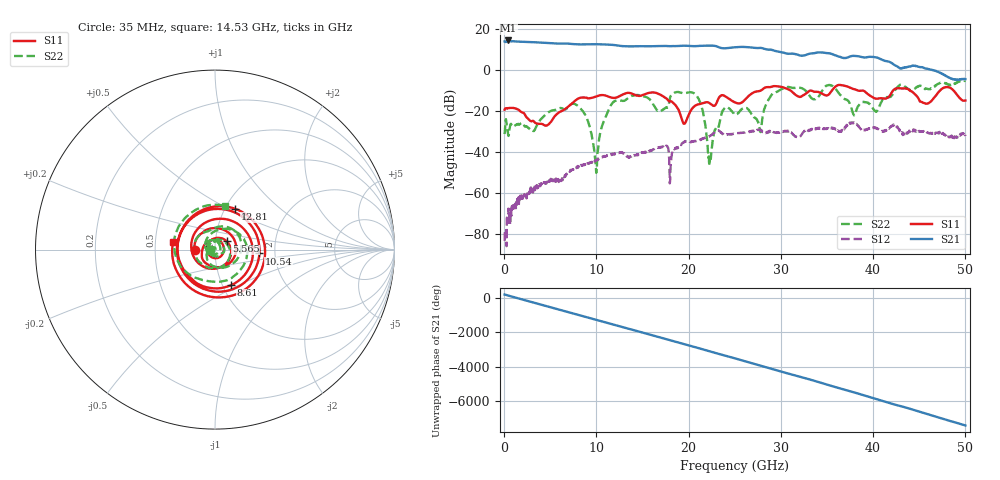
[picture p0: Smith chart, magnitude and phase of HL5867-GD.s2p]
! 4/14/2021 8:59:28 AM
! H:\PRODUCTION_DATA\TEMP_S2P.S2P
! CHANNEL.1
! TR.MEASUREMENT
! CORRECTED.DATA
# GHZ S RI R 50.0
! FREQ.GHZ  S11RE  S11IM  S21RE  S21IM  S12RE  S12IM  S22RE  S22IM
!; PortSelection: Port_12
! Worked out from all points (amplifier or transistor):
!   1429 points, 35 MHz to 50.02 GHz, reference 50 ohm
!   highest |S21| = 14.6 dB at 420 MHz (marker M1)
!   |S21| within 3 dB of that: start of sweep to 23.12 GHz
!   unconditionally stable (mu >= 1): start of sweep to end of sweep
!   at 8.365 GHz: K = 22.97, MAG = 12.9 dB, |S12| = -46.4 dB
!   at 25.02 GHz: K = 4.65, MAG = 11.4 dB, |S12| = -30.8 dB
!   at 50.02 GHz: K = 21.93, MAG = -2.5 dB, |S12| = -32.1 dB
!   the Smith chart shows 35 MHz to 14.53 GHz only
!   S11 on the Smith chart (normalised r, x): 35 MHz: 0.80, +0.00; 5.565 GHz: 1.13, +0.11; 8.61 GHz: 1.10, -0.46; 10.54 GHz: 1.66, -0.08; 12.81 GHz: 1.12, +0.54; 14.53 GHz: 0.62, +0.05
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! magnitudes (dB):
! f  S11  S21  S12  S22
! 35 MHz  -19.3  14.1  -83.2  -31.1
! 420 MHz  -18.4  14.6  -74.4  -31.5
! 5.565 GHz  -22.0  13.1  -53.6  -19.2
! 8.365 GHz  -13.3  12.7  -46.4  -19.1
! 8.61 GHz  -13.2  12.7  -46.0  -20.5
! 9.905 GHz  -12.9  12.7  -44.0  -46.8
! 10.54 GHz  -12.1  12.7  -42.5  -28.3
! 12.81 GHz  -11.9  11.8  -40.3  -14.9
! 14.53 GHz  -12.5  11.7  -41.3  -12.1
! 16.7 GHz  -11.4  11.8  -37.9  -19.9
! 18.09 GHz  -15.1  11.8  -43.8  -12.2
! 19.5 GHz  -26.1  12.0  -34.9  -11.2
! 20.68 GHz  -17.3  11.8  -34.5  -11.6
! 22.3 GHz  -16.1  12.0  -32.0  -44.6
! 23.77 GHz  -12.2  10.8  -31.2  -19.3
! 25.02 GHz  -15.7  11.2  -30.8  -21.5
! 27.72 GHz  -10.1  10.9  -29.1  -29.1
! 29.3 GHz  -7.7  9.6  -30.3  -10.9
! 33.39 GHz  -10.1  8.2  -28.7  -13.8
! 37.94 GHz  -9.2  7.0  -25.7  -22.0
! 41.69 GHz  -13.1  4.2  -28.3  -13.1
! 50.02 GHz  -14.7  -4.3  -32.1  -5.1
